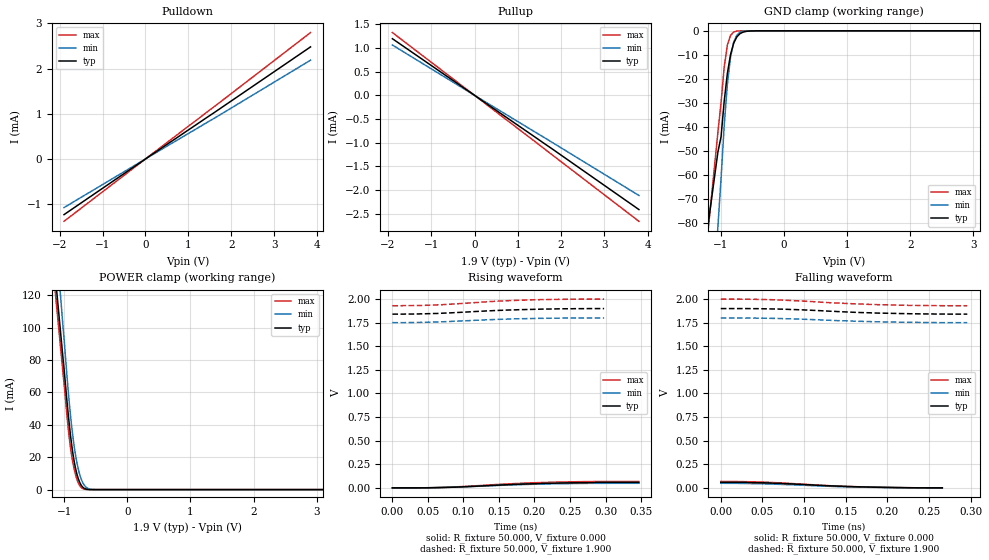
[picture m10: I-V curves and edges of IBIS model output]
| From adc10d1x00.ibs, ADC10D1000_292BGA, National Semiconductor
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[Model]   output
Model_type Output
Vref=0.000E+00
Rref=1.000E+06
Cref=0.000E+00
Vmeas=9.000E-01
C_comp   6.31E-13   6.31E-13   6.31E-13
[Voltage Range]   1.900E+00   1.800E+00   2.000E+00
[POWER Clamp Reference]   1.900E+00   1.800E+00   2.000E+00
[GND Clamp Reference]   0.000E+00   0.000E+00   0.000E+00
[Pullup Reference]   1.900E+00   1.800E+00   2.000E+00
[Pulldown Reference]   0.000E+00   0.000E+00   0.000E+00
[Temperature Range]   25   85   -40
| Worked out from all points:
|   slope of the pulldown table from 0 to 0.285 V, typ, clamps not added: 1.55 kohm
|   slope of the pullup table from 0 to 0.285 V, typ, clamps not added: 1.57 kohm
|   GND clamp passes 1 mA (typ) near -0.69 V on its own axis
|   POWER clamp passes 1 mA (typ) near -0.69 V on its own axis
|   rising waveform, R_fixture 50.000, V_fixture 0.000: 20-80 % time 109ps typ, NA min, 103ps max; typ from 0 V to 0.058 V
|   falling waveform, R_fixture 50.000, V_fixture 0.000: 20-80 % time 90.6ps typ, NA min, 91.2ps max; typ from 0.058 V to 0 V
|   rising waveform, R_fixture 50.000, V_fixture 1.900: 20-80 % time 105ps typ, NA min, 96ps max; typ from 1.84 V to 1.9 V
|   falling waveform, R_fixture 50.000, V_fixture 1.900: 20-80 % time 93.8ps typ, NA min, 98ps max; typ from 1.9 V to 1.84 V
[GND Clamp]
-1.9V     -216.2mA   -434.4mA   -266.5mA
-1.05V    -50.53mA   -81.7mA    -42.27mA
-1V       -44.21mA   -61.67mA   -29.97mA
-950mV    -29.35mA   -39.51mA   -15.07mA
-900mV    -17.79mA   -22.38mA   -6.011mA
-850mV    -9.946mA   -11.09mA   -1.929mA
-800mV    -5.178mA   -4.772mA   -503uA
-750mV    -2.538mA   -1.79mA    -107.5uA
-700mV    -1.183mA   -593.4uA   -18.49uA
-600mV    -228.6uA   -50.37uA   -1.511uA
-500mV    -38.34uA   -3.373uA   -939nA
3.8V      0A         0A         0A
[Power Clamp]
-1.9V     445.6mA    521.6mA    430.3mA
-1.02V    80.8mA     100.5mA    71.56mA
-960mV    55.46mA    71.25mA    46.5mA
-920mV    39.82mA    53.13mA    31.44mA
-860mV    21.28mA    31.49mA    15.64mA
-820mV    12.76mA    20.85mA    8.872mA
-780mV    6.911mA    12.9mA     4.233mA
-740mV    3.237mA    7.338mA    1.604mA
-700mV    1.238mA    3.749mA    453.3uA
-640mV    186.5uA    1.048mA    45.96uA
-520mV    1.547uA    31.18uA    305.9nA
3.8V      0A         0A         0A
[Pullup]
-1.9V     1.197mA    1.063mA    1.326mA
60mV      -38.49uA   -33.68uA   -40.26uA
1.76V     -1.11mA    -974.8uA   -1.233mA
3.8V      -2.413mA   -2.115mA   -2.661mA
[Pulldown]
-1.9V     -1.232mA   -1.075mA   -1.379mA
100mV     65.4uA     58.72uA    74.62uA
1.65V     1.056mA    926.5uA    1.192mA
3.85V     2.48mA     2.187mA    2.797mA
[Rising Waveform]
R_fixture = 50.000
V_fixture = 0.000
V_fixture_min = 0.000
V_fixture_max = 0.000
|  time   V(typ)   V(min)   V(max)
0s        493.4nV    928.3nV    -1.216uV
41ps      42.34uV    628.1uV    483.7uV
73ps      4.081mV    4.588mV    5.652mV
93ps      8.866mV    8.752mV    11.75mV
147ps     28.11mV    25.12mV    35.77mV
183ps     39.79mV    34.77mV    49.12mV
199ps     43.86mV    38.21mV    53.97mV
228ps     49.73mV    43.01mV    60.24mV
273ps     55.62mV    47.29mV    66.19mV
347ps     58.1mV     48.5mV     67.69mV
[Falling Waveform]
R_fixture = 50.000
V_fixture = 0.000
V_fixture_min = 0.000
V_fixture_max = 0.000
|  time   V(typ)   V(min)   V(max)
0s        58.1mV     48.5mV     67.69mV
25ps      57.24mV    46.92mV    66.23mV
54ps      52.44mV    42.1mV     59.72mV
82ps      42.81mV    33.47mV    47.66mV
119ps     26.38mV    20.24mV    28.09mV
131ps     21.61mV    16.21mV    22.71mV
165ps     11.06mV    7.992mV    11.77mV
218ps     2.261mV    1.422mV    2.615mV
244ps     134.2uV    75.17uV    493.5uV
266ps     493.6nV    929.6nV    -1.216uV
[Rising Waveform]
R_fixture = 50.000
V_fixture = 1.900
V_fixture_min = 1.800
V_fixture_max = 2.000
|  time   V(typ)   V(min)   V(max)
0s        1.841V     1.751V     1.93V
36ps      1.843V     1.753V     1.932V
55ps      1.846V     1.756V     1.936V
68ps      1.85V      1.759V     1.94V
146ps     1.879V     1.785V     1.978V
157ps     1.883V     1.788V     1.982V
194ps     1.891V     1.794V     1.992V
232ps     1.897V     1.798V     1.997V
259ps     1.899V     1.8V       2V
298ps     1.9V       1.8V       2V
[Falling Waveform]
R_fixture = 50.000
V_fixture = 1.900
V_fixture_min = 1.800
V_fixture_max = 2.000
|  time   V(typ)   V(min)   V(max)
0s        1.9V       1.8V       2V
23ps      1.9V       1.8V       2V
47ps      1.899V     1.798V     1.997V
61ps      1.896V     1.796V     1.994V
99ps      1.886V     1.787V     1.979V
140ps     1.868V     1.772V     1.958V
189ps     1.852V     1.76V      1.941V
223ps     1.846V     1.754V     1.935V
254ps     1.843V     1.752V     1.931V
296ps     1.841V     1.751V     1.93V
[Ramp]
dV/dt_r 32.7473m/151.129p 26.9891m/143.575p 38.1376m/133.420p
dV/dt_f 33.3468m/95.4672p 27.5419m/97.4521p 39.3908m/96.4084p
R_load = 50
